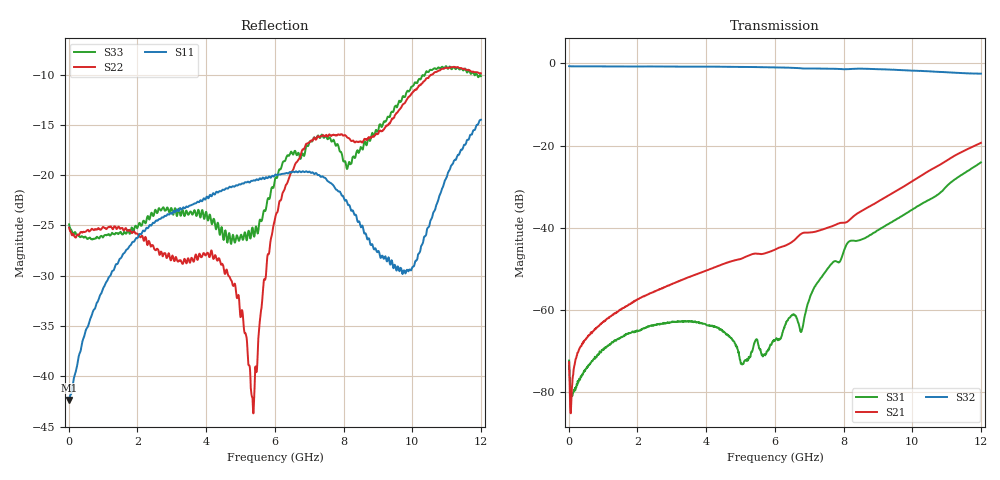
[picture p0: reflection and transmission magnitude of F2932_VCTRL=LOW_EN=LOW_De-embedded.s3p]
! Integrated Device Technology
! Corporate Headquarters
! 6024 Silver Creek Valley Road
! San Jose, CA 95138  USA
! Phone:  1-408-284-8200
! Toll Free:  1-800-223-1366
! Webpage:  http://www.idt.com/
! Timing and RF Division
! 515 Groton Road, Suite 102
! Westford, MA 01886-6024
! Device:  F2932
! Description: High Reliability SP2T RF Switch
! Frequency:  0.05 -  8.00 GHz
! Package:  4x4 mm QFN Plastic Package: 16 pin
! Ports:  3 RF, 3 DC
!  Pin  1  = VDD
!  Pin  2  = VCTL
!  Pin  3  = RFC  =  Port 3
!  Pin  4  = GND
!  Pin  5  = EN
!  Pin  6  = GND
!  Pin  7  = GND
!  Pin  8  = GND
!  Pin  9  = RF1  =  Port 1
!  Pin 10  = GND
!  Pin 11  = GND
!  Pin  9  = RF2  =  Port 2
!  Pin 13  = GND
!  Pin 14  = GND
!  Pin 15  = GND
!  Pin 16  = NC
! State:  RF2 Selected.
! VCTRL:  +0.00 Volts (Logic Low)
! EN:  +0.00 Volts (Logic Low)
! Voltage:  +5.00 Volts
! Current:  0.404 mA
! Data:  The device was measured on a F2932 evaluation board which has
!  individual transmission lines to the RF pins.  Data was collected
!  using a calibrated network analyzer.  The evaluation board was
!  de-embedded using AFR (Keysight) technique.
!  The reference plane is the edge of the package pin.
! Misc:
!  Action Tracker AT0443
! Date Measured:  2018-10-10
! Date:  2018-10-11  MJV
! Note:
!  Integrated Device Technology supplies this data as a sample of measured
!  data at the package pin for this product.  Your particular data for this
!  product may vary.
!  Data was taken at 25 degrees C.
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# Hz S dB R 50
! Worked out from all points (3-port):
!   1200 points, 10 MHz to 12 GHz, reference 50 ohm
!   strongest paths, dB at 10 MHz, 3.01 GHz, 6.01 GHz, 9.01 GHz, 12 GHz:
!     S32: -0.7, -0.8, -1.0, -1.4, -2.5
!     S21: -72.7, -53.7, -45.3, -33.6, -19.3
!     S31: -72.3, -62.8, -67.3, -40.5, -24.1
!   lowest |S11| = -42.4 dB at 10 MHz (marker M1), VSWR 1.02, Z = 49.2 - j0.000574 ohm
!   |S11| at or under -10 dB: start of sweep to end of sweep
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1e7  -42.35 -180.0  -72.12 -8.5  -72.46 -19.0
     -72.68 -8.7  -25.21 -3.3  -0.65 -0.4
     -72.30 -19.6  -0.66 -0.4  -24.89 -3.0
1.3e8  -40.58 124.9  -75.57 63.6  -79.88 -132.7
       -75.65 64.0  -25.82 -5.1  -0.70 -2.5
       -80.03 -136.3  -0.70 -2.5  -25.88 -3.5
1.62e9  -27.73 56.3  -59.33 77.7  -66.22 95.7
        -59.33 78.2  -25.44 -21.1  -0.73 -29.6
        -66.08 95.7  -0.73 -29.6  -25.65 -28.7
4.32e9  -21.68 20.6  -49.38 87.7  -64.47 23.3
        -49.37 88.0  -28.47 -38.3  -0.79 -79.1
        -64.21 22.9  -0.79 -79.1  -24.90 -64.1
5.35e9  -20.57 3.6  -46.40 86.2  -70.29 2.6
        -46.38 86.4  -42.18 -139.4  -0.87 -98.5
        -69.87 1.3  -0.87 -98.5  -25.20 -112.7
6.01e9  -19.95 -8.4  -45.26 91.1  -67.64 -157.0
        -45.28 91.3  -24.23 134.0  -0.96 -111.2
        -67.33 -161.4  -0.97 -111.1  -20.33 -159.6
6.78e9  -19.68 -19.2  -41.40 93.6  -65.01 15.5
        -41.39 93.9  -17.65 115.5  -1.22 -126.2
        -64.97 18.2  -1.22 -126.2  -18.06 -172.9
8.14e9  -22.98 -40.3  -38.33 94.7  -43.50 -159.8
        -38.34 94.8  -16.29 92.1  -1.39 -150.4
        -43.48 -159.2  -1.38 -150.4  -18.96 157.9
9.77e9  -29.49 -155.4  -29.85 82.0  -36.72 162.4
        -29.87 82.3  -12.87 52.1  -1.67 176.3
        -36.78 162.8  -1.65 176.4  -12.23 109.2
1.2e10  -14.48 87.5  -19.35 20.9  -23.99 106.3
        -19.33 21.4  -9.86 17.6  -2.46 131.1
        -24.08 106.9  -2.48 131.2  -10.14 76.7
